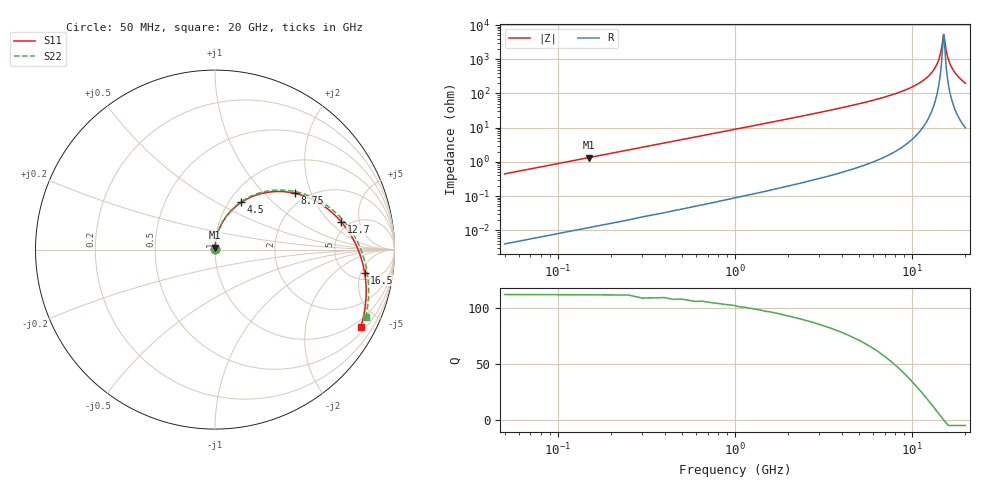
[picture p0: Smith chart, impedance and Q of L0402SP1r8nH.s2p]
!	AVX Thin Film Operation
!	Date:		5 January 2004
!	Description: 	Accu-L®  L0402 Series Thin Film RF Inductors
!	Part Number:	L04021R8AHLTR
!	50 MHz-20GHz Serial Measurements
#	mhz	S	db	R	50
!	S11	S11	S21	S21	S12	S12	S22	S22
!	dB	Phase	dB	Phase	dB	Phase	dB	Phase
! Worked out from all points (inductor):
!   400 points, 50 MHz to 20 GHz, reference 50 ohm
!   read as 1/Y11, port 2 shorted: L = 1.41 nH near 150 MHz
!   highest Q = 111 at 150 MHz (marker M1), where L = 1.41 nH
!   self-resonance near 15.05 GHz
!   S11 on the Smith chart (normalised r, x): 50 MHz: 1.00, +0.01; 4.5 GHz: 1.14, +0.66; 8.75 GHz: 1.74, +1.55; 12.7 GHz: 4.33, +2.77; 16.5 GHz: 6.54, -5.81; 20 GHz: 0.70, -3.90
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50  -49.27 89.0  -0.00 -0.3  -0.00 -0.3  -49.27 89.0
100  -43.25 88.7  -0.00 -0.6  -0.00 -0.6  -43.25 88.7
150  -39.73 88.4  -0.00 -0.9  -0.00 -0.9  -39.73 88.4
250  -35.29 87.7  -0.00 -1.6  -0.00 -1.6  -35.29 87.8
350  -32.37 87.1  -0.01 -2.2  -0.01 -2.2  -32.37 87.2
450  -30.19 86.5  -0.01 -2.8  -0.01 -2.8  -30.19 86.5
700  -26.35 84.9  -0.02 -4.4  -0.02 -4.4  -26.35 85.0
1050  -22.83 82.6  -0.03 -6.5  -0.03 -6.5  -22.83 82.8
1450  -20.04 80.1  -0.05 -9.0  -0.05 -9.0  -20.04 80.3
2000  -17.27 76.6  -0.10 -12.5  -0.10 -12.5  -17.27 76.9
2650  -14.86 72.5  -0.17 -16.5  -0.17 -16.5  -14.86 72.9
3400  -12.75 67.7  -0.27 -21.1  -0.27 -21.1  -12.75 68.3
4500  -10.42 60.9  -0.46 -27.8  -0.46 -27.8  -10.42 61.6
6700  -7.24 47.3  -0.98 -41.1  -0.98 -41.1  -7.24 48.5
8750  -5.26 35.0  -1.65 -53.0  -1.65 -53.0  -5.26 36.6
10050  -4.31 27.4  -2.16 -60.4  -2.16 -60.4  -4.31 29.2
12700  -2.84 12.3  -3.44 -75.0  -3.44 -75.0  -2.84 14.5
13350  -2.56 8.6  -3.80 -78.5  -3.80 -78.5  -2.56 11.0
16500  -1.48 -8.7  -5.98 -94.9  -5.98 -94.9  -1.48 -5.8
16700  -1.42 -9.8  -6.14 -95.9  -6.14 -95.9  -1.42 -6.8
18350  -1.03 -18.9  -7.69 -104.0  -7.69 -104.0  -1.03 -15.5
20000  -0.73 -27.9  -9.69 -111.7  -9.69 -111.7  -0.72 -24.2
